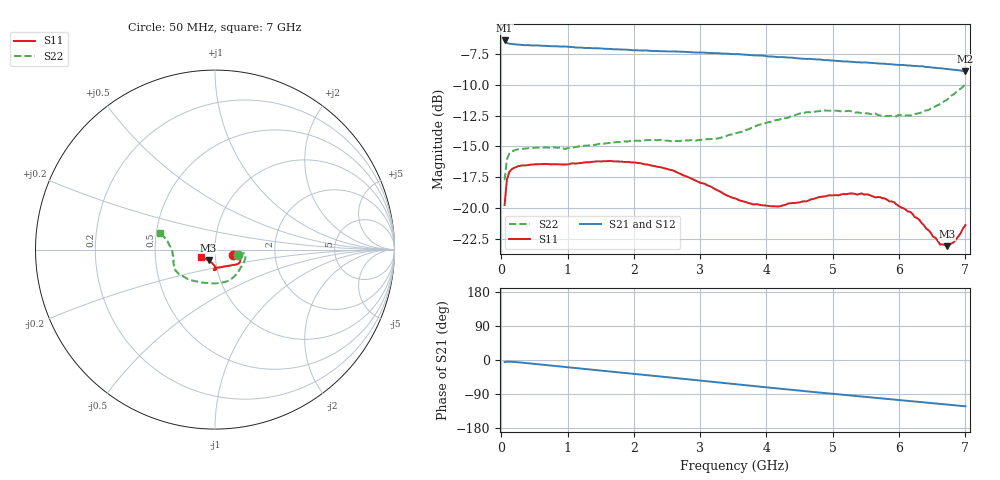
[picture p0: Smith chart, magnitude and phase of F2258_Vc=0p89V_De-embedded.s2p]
! Integrated Device Technology
! Corporate Headquarters
! 6024 Silver Creek Valley Road
! San Jose, CA 95138  USA
! Phone:  1-408-284-8200
! Toll Free:  1-800-223-1366
! Webpage:  http://www.idt.com/
! Timing and RF Division
! 515 Groton Road, Suite 102
! Westford, MA 01886-6024
! Device:  F2258
! Description: Voltage Variable RF Attenuator
! Frequency:  50.0 -  6000.00 MHz
! Package:  3x3 mm Thin QFN Plastic Package: 16 pin
! Ports:  2 RF, 2 DC
!  Pin  1  = NC
!  Pin  2  = NC
!  Pin  3  = RF2  = Port 2
!  Pin  4  = GND
!  Pin  5  = Vdd
!  Pin  6  = NC
!  Pin  7  = VCTRL
!  Pin  8  = NC
!  Pin  9  = GND
!  Pin 10  = RF1  = Port 1
!  Pin 11  = NC
!  Pin 12  = NC
!  Pin 13  = NC
!  Pin 14  = NC
!  Pin 15  = NC
!  Pin 16  = NC
! Vcntrl:  0.890 Volts
! Vdd:  +3.300 Volts
! Current:  1.145 mA
! Data:  The device was measured on a the F2258 evaluation board which has
!  individual transmission lines to the RF pins.  Data was collected
!  using a calibrated network analyzer.  The evaluation board was
!  de-embedded using a TRL calibration technique.
!  The reference plane is the edge of the package pin.
! Misc:  SN 10
!  Action Tracker AT0285
! Date Measured:  2014-12-10
! Date:  2016-01-13  MJV
! Note:
!  Integrated Device Technology supplies this data as a sample of measured
!  data at the package pin for this product.  Your particular data for this
!  product may vary.
!  Data was taken at 25 degrees C.
!  Integrated Device Technology reserves the right to change this data at anytime.
!Freq_(GHz)  S11M_(dB)  S11P_(deg)  S21M_(dB)  S21P_(deg)  S12M_(dB)  S12P_(deg)  S22M_(dB)  S22P_(deg)
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# GHz S dB R 50
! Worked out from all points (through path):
!   201 points, 50 MHz to 7 GHz, reference 50 ohm
!   highest |S21| = -6.39 dB at 50 MHz (marker M1); lowest = -8.9 dB at 7 GHz (marker M2)
!   group delay of S21, straight-line fit = 48.1 ps
!   lowest |S11| = -23.1 dB at 6.722 GHz (marker M3), VSWR 1.15, Z = 46.2 - j5.59 ohm
!   |S11| at or under -10 dB: start of sweep to end of sweep
!   |S22| runs from -17.7 to -9.9 dB; largest |S21 - S12| = 0.0024
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0.05  -19.76 -17.9  -6.39 -5.5  -6.42 -5.6  -17.75 -12.9
0.08475  -17.70 -8.9  -6.59 -4.5  -6.59 -4.5  -16.05 -7.8
0.1195  -17.10 -6.6  -6.66 -4.4  -6.65 -4.4  -15.59 -7.4
0.189  -16.76 -6.0  -6.70 -5.1  -6.72 -5.1  -15.34 -8.6
0.6755  -16.43 -13.3  -6.82 -13.3  -6.83 -13.3  -15.08 -23.5
0.9535  -16.47 -19.2  -6.88 -18.3  -6.88 -18.3  -15.22 -33.3
1.2315  -16.33 -22.7  -6.98 -23.2  -6.96 -23.2  -14.96 -42.0
1.6485  -16.18 -27.4  -7.08 -30.5  -7.06 -30.5  -14.71 -53.8
2.37825  -16.67 -33.7  -7.26 -43.2  -7.24 -43.2  -14.48 -73.7
2.93425  -17.77 -41.8  -7.37 -53.0  -7.33 -53.1  -14.53 -92.1
3.525  -19.22 -59.2  -7.51 -63.7  -7.48 -63.7  -13.96 -115.4
3.803  -19.72 -70.6  -7.60 -68.7  -7.57 -68.7  -13.41 -125.9
4.1505  -19.88 -82.0  -7.73 -74.8  -7.70 -74.8  -12.85 -136.3
4.7065  -19.27 -92.3  -7.91 -84.3  -7.93 -84.3  -12.21 -149.1
5.2625  -18.83 -92.3  -8.12 -93.5  -8.15 -93.5  -12.12 -158.1
5.43625  -18.82 -90.2  -8.18 -96.4  -8.18 -96.4  -12.30 -161.0
5.85325  -19.47 -87.5  -8.31 -103.2  -8.27 -103.3  -12.52 -169.6
6.166  -20.31 -89.1  -8.42 -108.4  -8.41 -108.4  -12.50 -176.8
6.61775  -22.98 -110.1  -8.65 -115.9  -8.63 -115.9  -11.56 171.2
6.722  -23.11 -120.7  -8.71 -117.7  -8.67 -117.7  -11.22 168.4
6.82625  -22.79 -132.7  -8.77 -119.3  -8.74 -119.4  -10.76 166.5
7  -21.40 -152.4  -8.89 -122.1  -8.88 -122.1  -9.95 163.0
